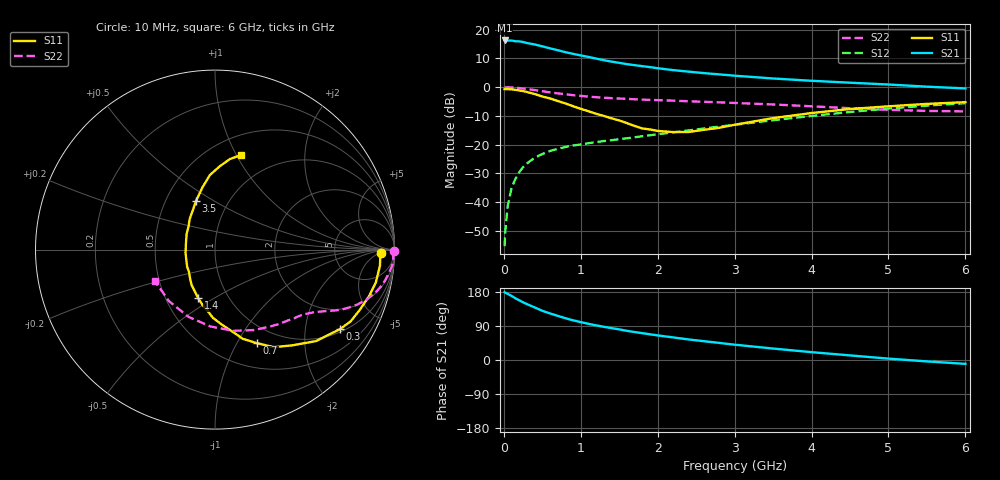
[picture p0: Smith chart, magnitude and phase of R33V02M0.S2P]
! SIEMENS Small Signal Semiconductors
! BFR181
! Si NPN RF Bipolar Junction Transistor in SOT23
! VCE = 3 V  IC = 2 mA
! Common Emitter S-Parameters:  May  1996
# GHz  S  MA  R  50
!  f  S11  S21  S12  S22
! GHz  MAG  ANG  MAG  ANG  MAG  ANG  MAG  ANG
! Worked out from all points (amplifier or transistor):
!   36 points, 10 MHz to 6 GHz, reference 50 ohm
!   highest |S21| = 16.3 dB at 10 MHz (marker M1)
!   |S21| within 3 dB of that: start of sweep to 639.7 MHz
!   unconditionally stable (mu >= 1): 1.589 GHz to 3.373 GHz
!   at 250 MHz: K = 0.23, MSG = 21.8 dB, |S12| = -27.9 dB
!   at 1.4 GHz: K = 0.95, MSG = 13.7 dB, |S12| = -18.5 dB
!   at 6 GHz: K = 0.86, MSG = 2.6 dB, |S12| = -5.6 dB
!   lowest NFmin = 1.35 dB at 450 MHz
!   S11 on the Smith chart (normalised r, x): 10 MHz: 24, -6; 300 MHz: 1.10, -3.06; 700 MHz: 0.78, -1.22; 1.4 GHz: 0.72, -0.43; 3.5 GHz: 0.71, +0.41; 6 GHz: 0.70, +1.05
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0.01  0.9247 -1.2  6.503 179.0  0.0017 94.2  0.9968 -0.6
0.02  0.9218 -2.4  6.362 177.6  0.0032 90.9  0.9911 -1.1
0.05  0.9235 -5.6  6.482 174.5  0.0085 87.2  0.9946 -2.7
0.1  0.9146 -11.5  6.491 169.1  0.0174 83.2  0.9902 -5.3
0.15  0.8969 -16.8  6.298 162.8  0.0252 79.6  0.9768 -7.9
0.2  0.8747 -22.4  6.27 157.6  0.0329 76.9  0.9633 -10.3
0.25  0.8549 -27.9  6.115 152.3  0.0404 73.5  0.9465 -12.6
0.3  0.8246 -32.6  5.862 147.5  0.0469 71.3  0.9286 -14.6
0.4  0.7589 -42.2  5.545 138.8  0.0589 66.3  0.8904 -18.2
0.5  0.6862 -51.0  5.132 129.8  0.0684 62.4  0.8488 -21.2
0.7  0.5728 -65.7  4.399 116.5  0.0842 57.5  0.7796 -25.4
0.8  0.5205 -72.7  4.064 110.3  0.0906 55.5  0.7513 -26.8
0.9  0.4656 -78.2  3.799 104.7  0.0963 54.4  0.725 -28.1
1.1  0.3799 -91.8  3.355 95.5  0.1056 53.4  0.684 -30.3
1.4  0.2861 -109.1  2.782 84.0  0.1191 53.2  0.6433 -33.2
1.8  0.1909 -139.3  2.319 70.8  0.1397 54.5  0.6065 -36.8
2.2  0.1651 -173.8  1.98 59.6  0.163 55.4  0.5817 -41.6
2.8  0.1961 138.8  1.669 45.1  0.2059 55.8  0.5436 -50.0
3.5  0.2891 111.6  1.415 30.2  0.2652 53.2  0.4991 -63.9
4.5  0.4164 93.9  1.195 12.1  0.3694 45.1  0.429 -93.3
5.5  0.511 80.7  1.019 -3.7  0.4767 32.6  0.3853 -131.6
6  0.5476 74.5  0.95 -10.2  0.5253 25.3  0.3784 -152.2
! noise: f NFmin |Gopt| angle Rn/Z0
0.45  1.35  0.6  17  0.4
0.9  1.45  0.5  36  0.4
1.8  1.8  0.31  80  0.37
